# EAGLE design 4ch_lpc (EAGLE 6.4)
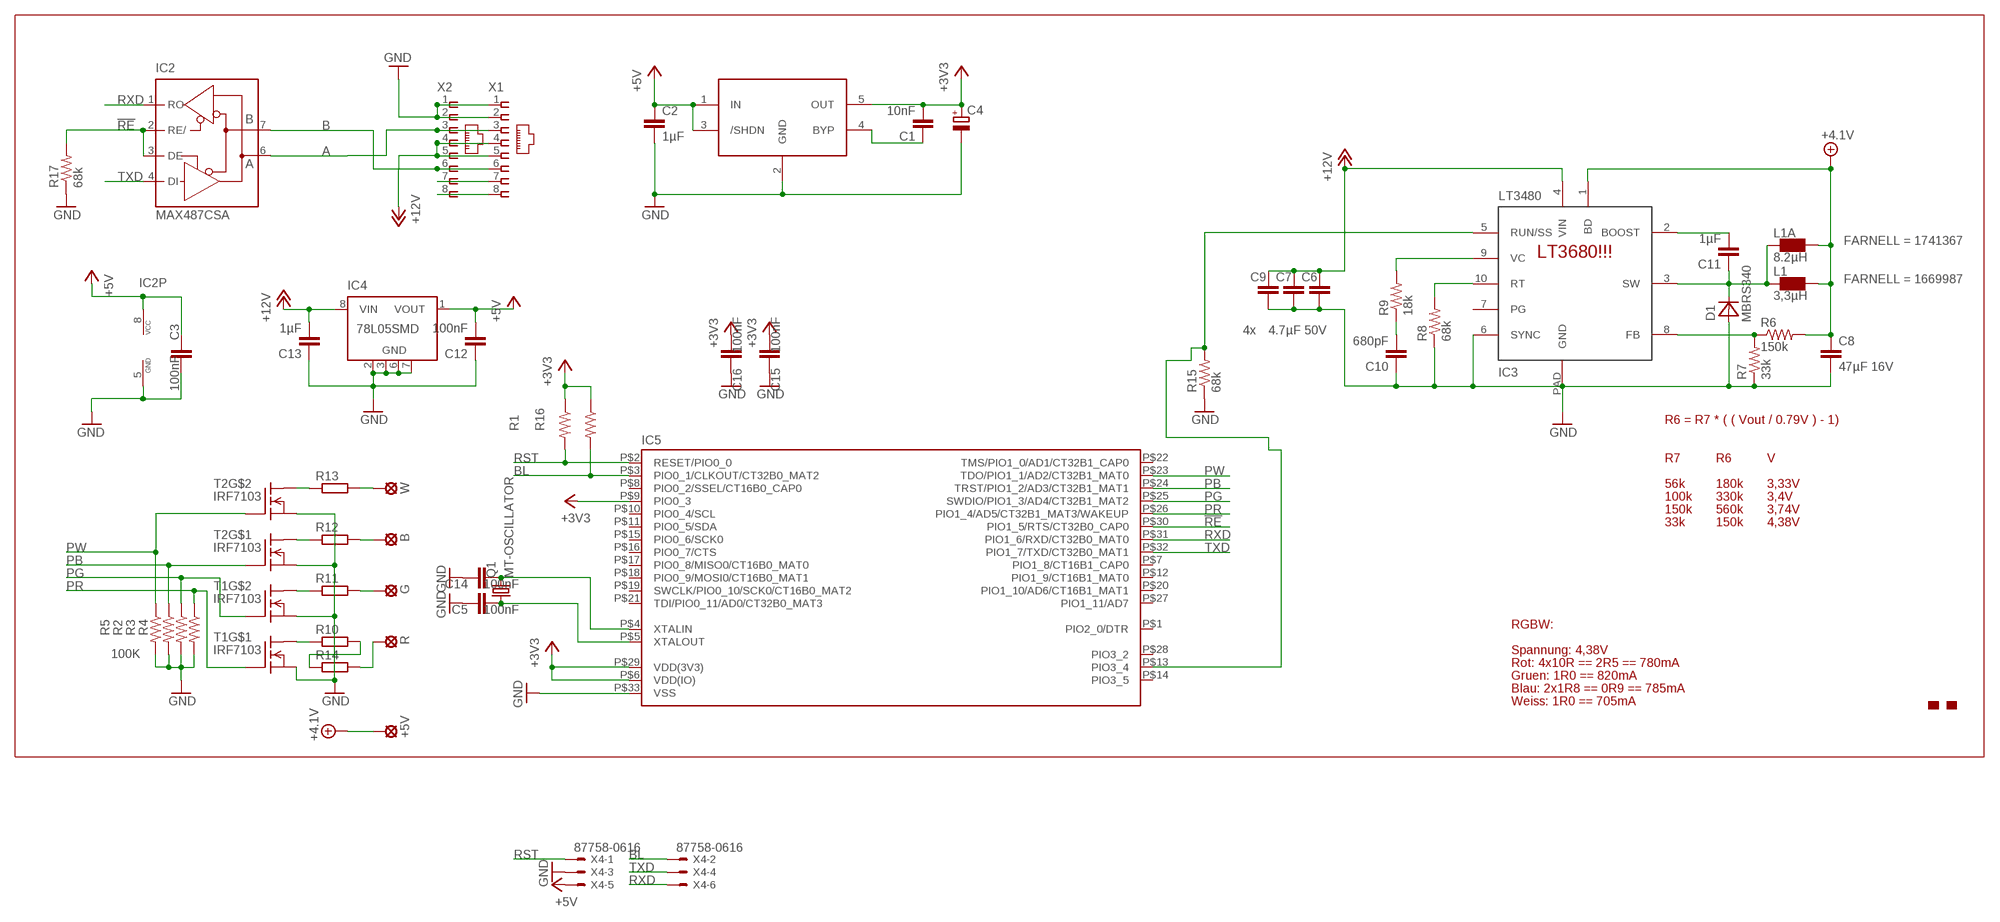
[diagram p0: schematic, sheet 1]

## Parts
+5V  SE14  [SE14]
B  SE14  [SE14]
C1  10nF  C-EUC0402  [C0402]
C2  1µF  CAP0805  [0805]
C3  100nF  CAP0402-CAP  [0402-CAP]
C4  CPOL-EUSMCA  [SMC_A]
C5  100nF  CAP0402-CAP  [0402-CAP]
C6  4.7µF 50V  CAP1210  [1210]
C7  4.7µF 50V  CAP1210  [1210]
C8  47µF 16V  CAP1210  [1210]
C9  4.7µF 50V  CAP1210  [1210]
C10  680pF  CAP0805  [0805]
C11  1µF  CAP0805  [0805]
C12  100nF  CAP0402-CAP  [0402-CAP]
C13  1µF  CAP0805  [0805]
C14  100nF  CAP0402-CAP  [0402-CAP]
C15  100nF  CAP0402-CAP  [0402-CAP]
C16  100nF  CAP0402-CAP  [0402-CAP]
D1  MBRS340  [DO214AB]
G  SE14  [SE14]
IC1  LT1761  [SOT23-5L]
IC2  MAX487CSA  MAX481CSA  [SO08]
IC3  LT3972  LT3480  [MSOP10-PAD]
IC4  78L05SMD  [SO08]
IC5  LPC1113/4_QFN  [HVQFN33-7X7]
L1  3,3µH  TDK_RLF7030  [RLF7030]
L1A  8.2µH  IHLP-2525CZ  [IHLP-2525CZ]
Q1  MT-OSCILLATOR  [MT]
R  SE14  [SE14]
R1  100K  RESISTOR0402-RES  [0402-RES]
R2  100K  RESISTOR0402-RES  [0402-RES]
R3  100K  RESISTOR0402-RES  [0402-RES]
R4  100K  RESISTOR0402-RES  [0402-RES]
R5  100K  RESISTOR0402-RES  [0402-RES]
R6  150k  RESISTOR0805-RES  [0805]
R7  33k  RESISTOR0805-RES  [0805]
R8  68k  RESISTOR0805-RES  [0805]
R9  18k  RESISTOR0805-RES  [0805]
R10  R-EU_MELF0207R  [MINI_MELF-0207R]
R11  R-EU_MELF0207R  [MINI_MELF-0207R]
R12  R-EU_MELF0207R  [MINI_MELF-0207R]
R13  R-EU_MELF0207R  [MINI_MELF-0207R]
R14  R-EU_MELF0207R  [MINI_MELF-0207R]
R15  68k  RESISTOR0402-RES  [0402-RES]
R16  100K  RESISTOR0402-RES  [0402-RES]
R17  68k  RESISTOR0402-RES  [0402-RES]
T1  IRF7103  [SO-8]
T2  IRF7103  [SO-8]
U$1  MAKE-DD_LOGO'PROMPT'  [MAKE-DD_LOGO_PROMPT]
W  SE14  [SE14]
X1  RJ45-8L-B  [RJ45-NO-SHIELD]
X2  RJ45-8L-B  [RJ45-NO-SHIELD]
X4  87758-0616  [87758-0616]

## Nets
!RE: IC2.2(RE/) IC2.3(DE) IC5.P$30(PIO1_5/RTS/CT32B0_CAP0) R17.2
+3V3: C1.2 C4.+ C15.2 C16.2 IC1.5(OUT) IC5.P$6(VDD(IO)) IC5.P$9(PIO0_3) IC5.P$29(VDD(3V3)) R1.1 R16.1
+4.1V: +5V.MP C8.1 IC3.1(BD) L1.P$1 L1A.P$1 R6.2
+5V: C2.1 C3.1 C12.2 IC1.1(IN) IC1.3(/SHDN) IC2.8(VCC) IC4.1(VOUT) X4.5
+12V: C6.1 C7.1 C9.1 C13.2 IC3.4(VIN) IC4.8(VIN) X1.4 X1.5 X2.4 X2.5
A: IC2.6(A) X1.3 X2.3
B: IC2.7(B) X1.6 X2.6
BL: IC5.P$3(PIO0_1/CLKOUT/CT32B0_MAT2) R16.2 X4.2
GND: C2.2 C3.2 C4.- C5.1 C6.2 C7.2 C8.2 C9.2 C10.1 C12.1 C13.1 C14.1 C15.1 C16.1 D1.A IC1.2(GND) IC2.5(GND) IC3.6(SYNC) IC3.PAD(GND) IC4.2(GND) IC4.3(GND) IC4.6(GND) IC4.7(GND) IC5.P$33(VSS) R2.2 R3.2 R4.2 R5.2 R7.1 R8.1 R15.1 R17.1 T1.1(S) T1.3(S) T2.1(S) T2.3(S) X1.1 X1.2 X2.1 X2.2 X4.3
N$1: R10.1 T1.8(D1)
N$2: R13.2 W.MP
N$3: R13.1 T2.5(D1)
N$4: R11.1 T1.5(D1)
N$5: R12.1 T2.8(D1)
N$6: IC3.10(RT) R8.2
N$7: C1.1 IC1.4(BYP)
N$8: G.MP R11.2
N$9: B.MP R12.2
N$10: C10.2 R9.1
N$11: R10.2 R14.1
N$12: IC3.5(RUN/SS) IC5.P$13(PIO3_4) R15.2
N$13: R14.2 R.MP
N$14: IC3.9(VC) R9.2
N$15: C11.1 D1.K(C) IC3.3(SW) L1.P$2 L1A.P$2
N$16: IC3.8(FB) R6.1 R7.2
N$17: C11.2 IC3.2(BOOST)
N$18: X1.7 X2.7
N$19: X1.8 X2.8
N$20: C5.2 IC5.P$5(XTALOUT) Q1.1
N$21: C14.2 IC5.P$4(XTALIN) Q1.3
PB: IC5.P$24(TRST/PIO1_2/AD3/CT32B1_MAT1) R2.1 T2.2(G)
PG: IC5.P$25(SWDIO/PIO1_3/AD4/CT32B1_MAT2) R3.1 T1.4(G)
PR: IC5.P$26(PIO1_4/AD5/CT32B1_MAT3/WAKEUP) R4.1 T1.2(G)
PW: IC5.P$23(TDO/PIO1_1/AD2/CT32B1_MAT0) R5.1 T2.4(G)
RST: IC5.P$2(RESET/PIO0_0) R1.2 X4.1
RXD: IC2.1(RO) IC5.P$31(PIO1_6/RXD/CT32B0_MAT0) X4.6
TXD: IC2.4(DI) IC5.P$32(PIO1_7/TXD/CT32B0_MAT1) X4.4
Unconnected: IC3.7(PG) IC4.4(NC) IC4.5(NC) IC5.P$1(PIO2_0/DTR) IC5.P$7(PIO1_8/CT16B1_CAP0) IC5.P$8(PIO0_2/SSEL/CT16B0_CAP0) IC5.P$10(PIO0_4/SCL) IC5.P$11(PIO0_5/SDA) IC5.P$12(PIO1_9/CT16B1_MAT0) IC5.P$14(PIO3_5) IC5.P$15(PIO0_6/SCK0) IC5.P$16(PIO0_7/CTS) IC5.P$17(PIO0_8/MISO0/CT16B0_MAT0) IC5.P$18(PIO0_9/MOSI0/CT16B0_MAT1) IC5.P$19(SWCLK/PIO0_10/SCK0/CT16B0_MAT2) IC5.P$20(PIO1_10/AD6/CT16B1_MAT1) IC5.P$21(TDI/PIO0_11/AD0/CT32B0_MAT3) IC5.P$22(TMS/PIO1_0/AD1/CT32B1_CAP0) IC5.P$27(PIO1_11/AD7) IC5.P$28(PIO3_2) T1.6(D) T1.7(D) T2.6(D) T2.7(D)

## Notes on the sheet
- LT3680!!!
- 4x
- R6 = R7 * ( ( Vout / 0.79V ) - 1)
- R7 | R6 | V
- 56k | 180k | 3,33V
- 100k | 330k | 3,4V
- 150k | 560k | 3,74V
- 33k | 150k | 4,38V
- RGBW:
- Spannung: 4,38V
- Rot: 4x10R == 2R5 == 780mA
- Gruen: 1R0 == 820mA
- Blau: 2x1R8 == 0R9 == 785mA
- Weiss: 1R0 == 705mA

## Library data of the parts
+5V B G R W = solpad:SE14: SOLDER PAD
C1 = rcl:C-EU: CAPACITOR, European symbol
C2 = SparkFun-Capacitors:CAP: Capacitor
C3 C5-C16 = SparkFun:CAP: Capacitor
C4 = rcl:CPOL-EU: POLARIZED CAPACITOR, European symbol
D1 = seb:MBRS340
IC1 = seb:LT1761
IC2 = maxim:MAX481CSA: RS485 TRANSEIVER; MF: MAXIM; MPN: MAX481CSA; OC_FARNELL: unknown; OC_NEWARK: 90C3817
IC3 = seb:LT3480
IC4 = linear:78L*SMD: Positive VOLTAGE REGULATOR
IC5 = microbuilder:LPC1113/4_QFN: LPC1113/4 ARM Cortex-M0 processor, running at frequencies of up to 50 MHz. QFN 33 Pin Package; DIGIKEY#: 568-4948-ND; MANF: NXP; MANF#: LPC1114FHN33/301,5
L1 = seb:TDK_RLF7030; FARNELL: 1669987
L1A = seb:IHLP-2525CZ; FARNELL: 1741367
Q1 = seb:MT-OSCILLATOR
R1-R9 R15-R17 = SparkFun:RESISTOR: Resistor
R10-R14 = rcl:R-EU_: RESISTOR, European symbol
T1 T2 = transistor-fet+irf7201:IRF7103
U$1 = seb:MAKE-DD_LOGO
X1 X2 = con-tycoelectronics:RJ45: CORCOM Modular RJ Jacks No Shield Source: www.tycoelectronics.com .. ENG_DS_1654001_1099_RJ_L_0507.pdf; MF: TYCO ELECTRONICS; MPN: RJ45-8L-B; OC_FARNELL: 1279843; OC_NEWARK: 52K4445
X4 = con-molex:87758-0616: 6 Pin - 2mm Dual Row Single Wafer, Vertical T/H HDR Source: http://www.molex.com/pdm_docs/sd/877580616_sd.pdf; MPN: 87758-0616; OC_FARNELL: 7472323; OC_NEWARK: 25M5667

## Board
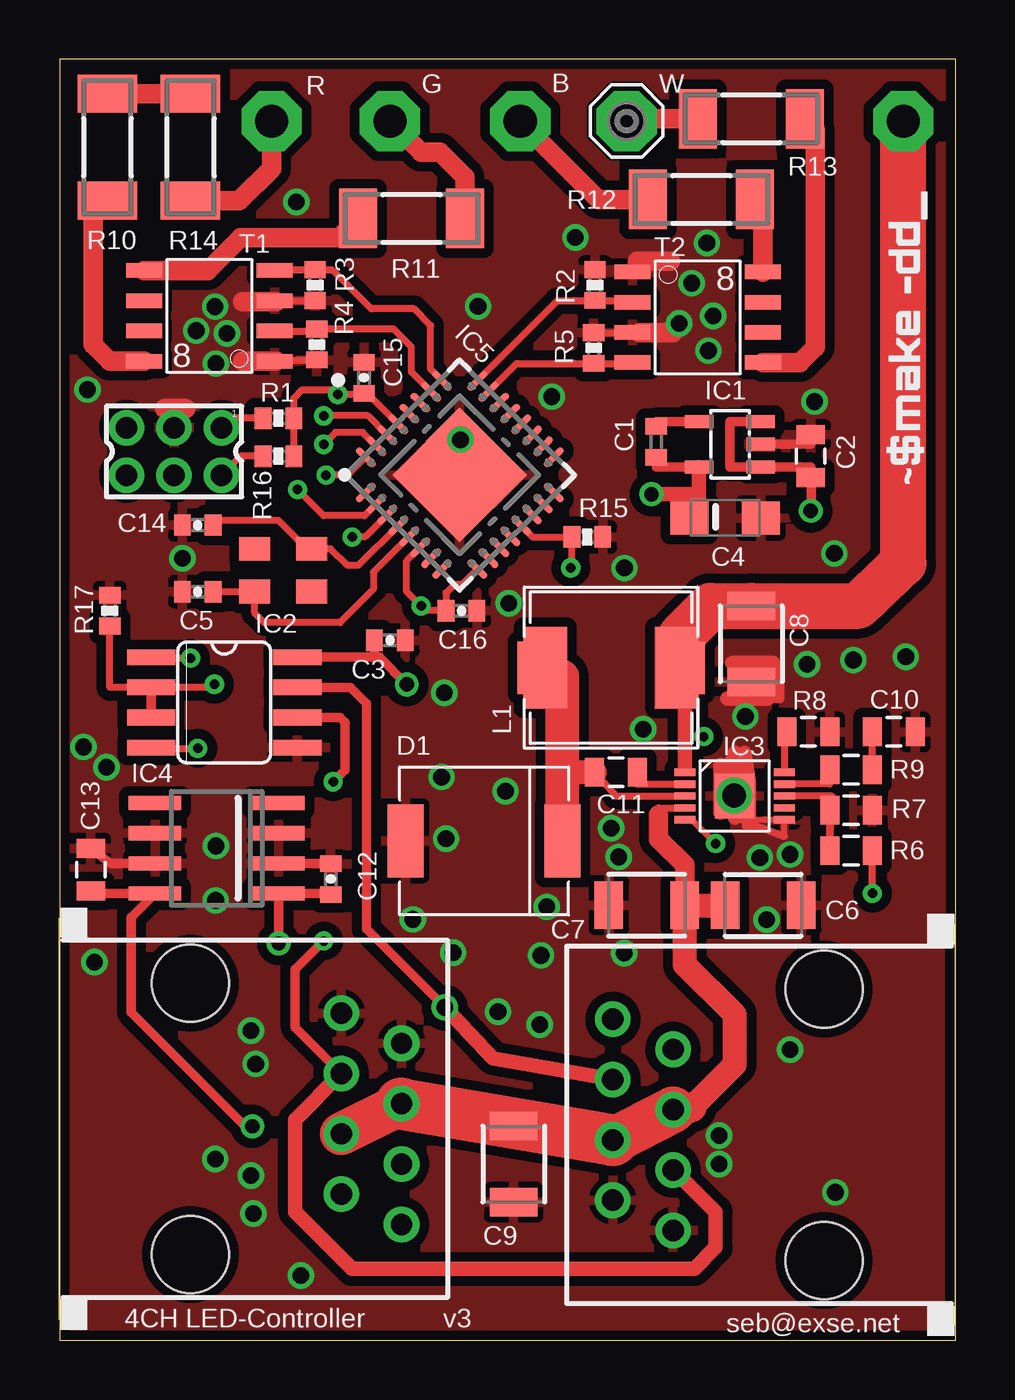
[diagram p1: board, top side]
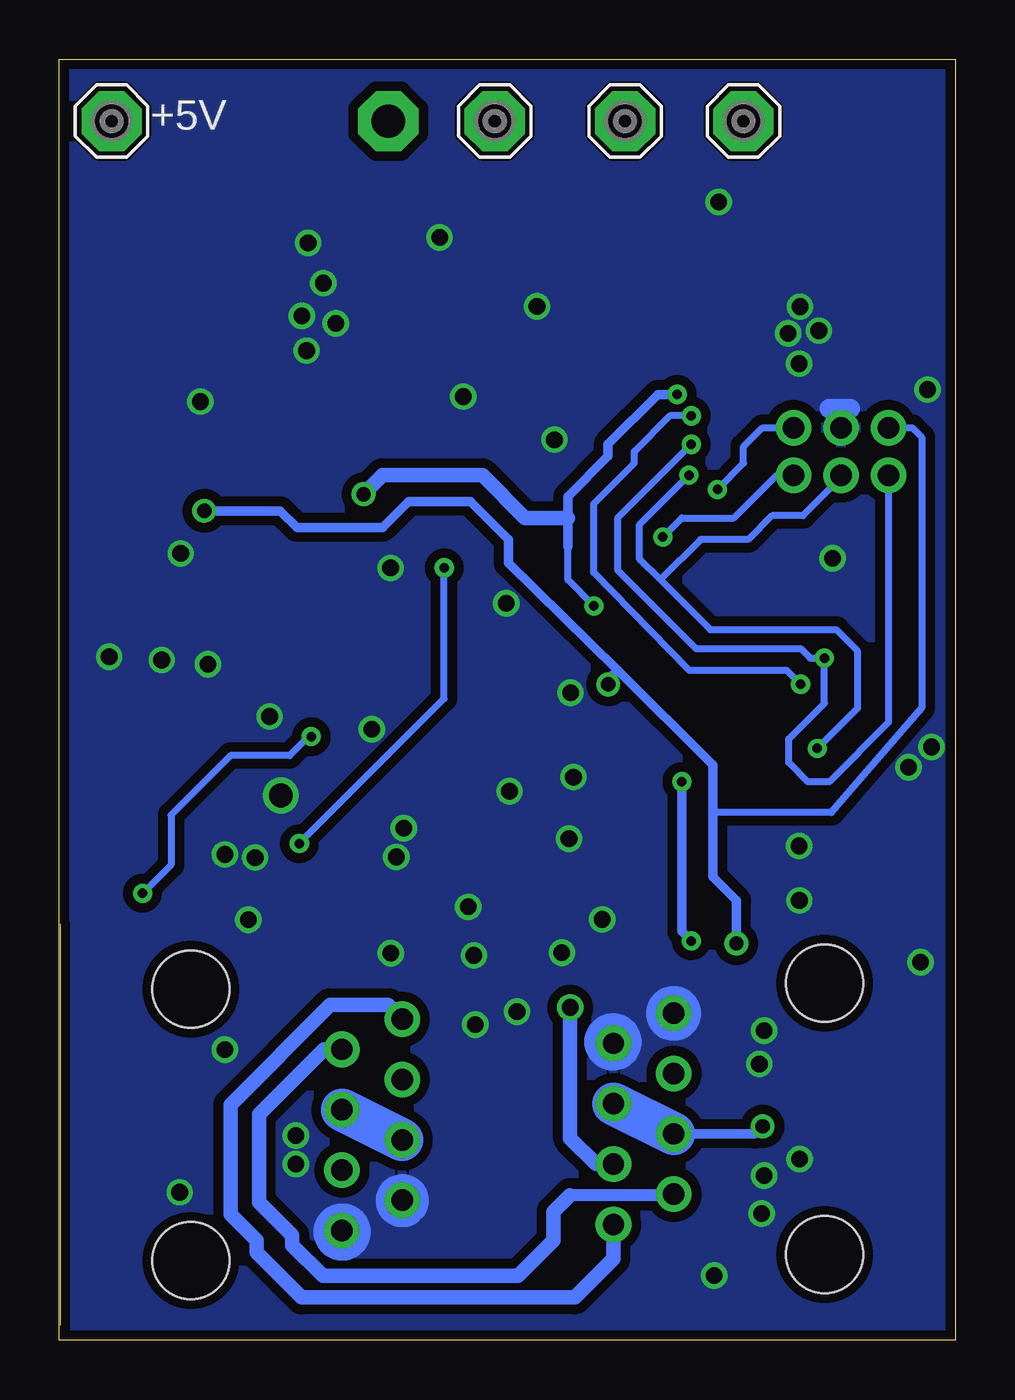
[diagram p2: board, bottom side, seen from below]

Size 37.72 x 53.9 mm. Coordinates in mm from the lower left corner, seen from the top.
Outline: 0.02,0 37.72,0 37.72,53.9 0.02,53.9 0.02,0
Copper layers (1*16): Top 0.035mm / dielectric 1.5mm / Bottom 0.035mm
Design rules "default *": minimum track width 0.2mm, minimum drill 0.4mm, track to track 0.2mm, track to pad 0.2mm, pad to pad 0.2mm, via to via 0.2mm, smd to smd 0mil, copper to edge 0.4mm, drill to drill 8mil, minimum pad ring 0.3mm, minimum via ring 8mil, stop-mask expansion 4mil, vias tented up to drill 40mil, thermal gap 10mil

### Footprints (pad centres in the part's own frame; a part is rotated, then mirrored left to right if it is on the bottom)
SE14 = drill 1.397 pad 2.54 octagon: MP 0,0
C0402 = smd 0.7 x 0.9: 1 -0.65,0; 2 0.65,0
0805 = smd 0.8 x 1.2: 1 -0.9,0; 2 0.9,0
0402-CAP = smd 0.7 x 0.9: 1 -0.65,0; 2 0.65,0
SMC_A = smd 1.6 x 1.4: + -1.5,0; - 1.5,0
1210 = smd 1.2 x 2: 1 -1.6,0; 2 1.6,0
DO214AB = smd 1.52 x 3.07: A 3.305,0; K -3.305,0
SOT23-5L = smd 0.55 x 1.2: 1 -0.95,-1.3; 2 0,-1.3; 3 0.95,-1.3; 4 0.95,1.3; 5 -0.95,1.3
SO08 = smd 0.66 x 2.032: 1 -1.905,-3.073; 2 -0.635,-3.073; 3 0.635,-3.073; 4 1.905,-3.073; 5 1.905,3.073; 6 0.635,3.073; 7 -0.635,3.073; 8 -1.905,3.073
MSOP10-PAD = smd 0.305 x 0.889: 1 -1,-2.095; 2 -0.5,-2.095; 3 0,-2.095; 4 0.5,-2.095; 5 1,-2.095; 6 1,2.095; 7 0.5,2.095; 8 0,2.095; 9 -0.5,2.095; 10 -1,2.095 | smd 1.88 x 1.68: PAD 0,0
SO08' = smd 0.6 x 2.2: 1 -1.905,-2.6; 2 -0.635,-2.6; 3 0.635,-2.6; 4 1.905,-2.6; 5 1.905,2.6; 6 0.635,2.6; 7 -0.635,2.6; 8 -1.905,2.6
HVQFN33-7X7 = smd 1.067 x 0.3: P$1 -3.327,2.275; P$2 -3.327,1.625; P$3 -3.327,0.975; P$4 -3.327,0.325; P$5 -3.327,-0.325; P$6 -3.327,-0.975; P$7 -3.327,-1.625; P$8 -3.327,-2.275; P$17 3.327,-2.275; P$18 3.327,-1.625; P$19 3.327,-0.975; P$20 3.327,-0.325; P$21 3.327,0.325; P$22 3.327,0.975; P$23 3.327,1.625; P$24 3.327,2.275 | smd 0.3 x 1.067: P$9 -2.275,-3.327; P$10 -1.625,-3.327; P$11 -0.975,-3.327; P$12 -0.325,-3.327; P$13 0.325,-3.327; P$14 0.975,-3.327; P$15 1.625,-3.327; P$16 2.275,-3.327; P$25 2.275,3.327; P$26 1.625,3.327; P$27 0.975,3.327; P$28 0.325,3.327; P$29 -0.325,3.327; P$30 -0.975,3.327; P$31 -1.625,3.327; P$32 -2.275,3.327 | smd 4 x 4: P$33 0,0
RLF7030 = smd 2 x 2.2: P$1 -2.95,0; P$2 2.95,0
IHLP-2525CZ = smd 1.83 x 3.43: P$1 -2.77,0; P$2 2.77,0
MT = smd 1.3 x 1: 1 1.2,0.9; 2 -1.2,0.9; 3 -1.2,-0.9; 4 1.2,-0.9
0402-RES = smd 0.7 x 0.9: 1 -0.65,0; 2 0.65,0
MINI_MELF-0207R = smd 1.6 x 2.5: 1 -2.25,0; 2 2.25,0
SO-8 = smd 1.524 x 0.61: 1 -2.743,1.27; 2 -2.743,0; 3 -2.743,-1.27; 4 -2.743,-2.54; 5 2.743,-2.54; 6 2.743,-1.27; 7 2.743,0; 8 2.743,1.27
RJ45-NO-SHIELD = drill 0.9 pad 1.4: 1 -4.445,6.35; 2 -3.175,8.89; 3 -1.905,6.35; 4 -0.635,8.89; 5 0.635,6.35; 6 1.905,8.89; 7 3.175,6.35; 8 4.445,8.89 | hole 3.251: -5.715,0; 5.715,0
87758-0616 = drill 0.9 pad 1.27: 1 -2,-1; 2 -2,1; 3 0,-1; 4 0,1; 5 2,-1; 6 2,1

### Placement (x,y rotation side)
+5V  35.52,51.3 0 bottom
B  19.39,51.3 0 bottom
C1  25.12,37.8 270 top
C2  31.62,37.2 90 top
C3  13.91,29.45 0 top
C4  28.02,34.6 0 top
C5  5.82,31.5 0 top
C6  29.62,18.3 0 top
C7  24.72,18.3 180 top
C8  29.12,29.3 270 top
C9  19.12,7.4 270 top
C10  35.12,25.6 180 top
C11  23.42,23.9 0 top
C12  11.42,19.4 270 top
C13  1.32,19.8 270 top
C14  5.82,34.3 0 top
C15  12.82,40.5 270 top
C16  16.92,30.7 180 top
D1  17.87,21.01 180 top
G  13.91,51.3 0 bottom
IC1  28.22,37.7 90 top
IC2  6.94,26.84 270 top
IC3  28.42,22.9 270 top
IC4  78L05SMD  [SO08']  6.62,20.7 90 top
IC5  16.85,36.41 45 top
L1  23.22,28.3 180 top
L1A  23.22,28.3 180 top
Q1  9.42,32.4 180 top
R  8.93,51.3 0 bottom
R1  9.22,38.8 180 top
R2  22.54,44.4 90 top
R3  10.76,44.4 270 top
R4  10.84,41.9 270 top
R5  22.49,41.75 90 top
R6  33.32,20.6 0 top
R7  33.32,22.3 180 top
R8  31.52,25.6 180 top
R9  33.32,24 180 top
R10  2.02,50.2 90 top
R11  14.82,47.2 0 top
R12  27.02,48 180 top
R13  29.12,51.4 180 top
R14  5.52,50.2 270 top
R15  22.22,33.8 180 top
R16  9.22,37.2 180 top
R17  2.12,30.7 270 top
T1  6.31,42.47 180 top
T2  26.87,43.68 0 top
U$1  36.22,36.2 90 top
W  23.88,51.3 0 top
X1  32.18,9.06 90 top
X2  5.51,9.31 270 top
X4  4.82,37.4 180 top

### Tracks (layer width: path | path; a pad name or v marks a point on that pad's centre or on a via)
!RE  (via drill 0.4)
  Top 0.3: IC5.P$30 12.99,38.9 v11.12,38.9
  Top 0.305: v6.52,27.6 6.39,27.47 IC2.2 2.12,27.47 R17.2
  Top 0.406: IC2.3 IC2.2
  Bottom 0.305: v11.12,38.9 12.02,38.9 13.52,37.4 13.52,36.9 15.22,35.2 15.22,32.3 11.22,28.2 7.12,28.2 v6.52,27.6
+3V3  (via drill 0.4, 0.6)
  Top 0.3: IC5.P$6 14.62,32.8 | IC5.P$29 12.95,39.85 C15.2 12.77,39.8 v11.72,39.8 | R16.1 R1.1
  Top 0.305: 14.62,32.8 14.62,31.5 v15.22,30.9 15.42,30.7 C16.2 16.27,31.45 16.62,31.8 16.94,31.8 IC5.P$9 | R1.1 9.87,39.65 10.22,40 11.52,40 v11.72,39.8
  Top 0.406: C1.2 25.12,36.75 IC1.5
  Top 0.61: IC1.5 26.92,35.5 | 26.92,35.5 26.92,34.4 C4.+ | v24.92,35.6 26.82,35.6 26.92,35.5
  Bottom 0.305: v15.22,30.9 16.32,32 16.32,33.4
  Bottom 0.406: v11.72,39.8 12.52,39.8 14.62,37.7 14.62,37.2 16.32,35.5 16.32,34.6 16.32,33.4
  Bottom 0.61: v24.92,35.6 24.12,36.4 19.92,36.4 18.12,34.6 16.32,34.6
+4.1V  (via drill 0.4)
  Top 0.254: L1.P$1 L1A.P$1
  Top 0.305: IC3.1 26.32,24.8 | v34.22,18.8 R6.2 | 26.32,25.4 v27.12,25.4
  Top 0.61: 26.32,24.1 26.32,24.8 26.32,25.4 26.32,27.9 L1.P$1
  Top 1.93: L1.P$1 26.17,29.65 27.42,30.9 C8.1 33.62,30.9 35.52,32.7 +5V.MP
  Bottom 0.305: v34.22,18.8 33.02,20 33.02,22.1 30.52,24.6 28.02,24.6 27.22,25.4 v27.12,25.4
+5V  (via drill 0.6)
  Top 0.406: C12.2 11.32,18.8 IC4.1 v9.22,16.7 | 13.22,28.74 13.48,28.74 v14.62,27.6 | 13.22,28.74 IC2.8 | v31.62,34.9 31.67,36.25 31.62,36.75 | 31.62,36.75 IC1.1 28.22,36.75 28.22,38.65 IC1.3 | C2.1 31.62,36.75 | C3.1 13.26,28.78 13.22,28.74
  Bottom 0.305: X4.5 1.82,38.4 1.42,38 1.42,26.6 5.22,22.2 10.22,22.2
  Bottom 0.406: v9.22,16.7 9.22,18.5 10.22,19.5 10.22,22.2 10.22,24.2 14.22,28.2 | 14.22,28.2 18.82,32.7 18.82,33.7 20.42,35.3 23.02,35.3 24.12,34.2 27.72,34.2 28.42,34.9 v31.62,34.9 | v14.62,27.6 14.62,27.8 14.22,28.2
+12V  (via drill 0.6)
  Top 0.3: IC3.4 25.22,22.4 25.22,22.1
  Top 0.406: v8.12,9 7.82,9 3.02,13.8 3.02,17.8 IC4.8 1.63,18.8 C13.2
  Top 0.813: 25.22,22.1 25.22,21.1 26.32,20 C7.1
  Top 1.016: 26.52,9.7 26.62,9.8 28.42,11.6 28.42,13.7 26.32,15.8 C7.1 C6.1 | C9.1 20.4,8.43 X1.4
  Top 1.27: X1.5 26.62,9.8
  Top 1.778: X2.5 X2.4
  Top 1.93: X1.5 23.32,8.4 X1.5
  Top 2.184: X2.4 X1.4
  Bottom 0.406: v8.12,9 8.44,8.68 X2.5
  Bottom 1.778: X1.4 X1.5 | X2.5 X2.4
A  (via drill 0.4)
  Top 0.406: IC2.6 11.82,26.2 12.02,26 12.02,24 v11.52,23.5 | X2.3 9.92,13.16 9.92,15.6 v11.12,16.8
  Top 0.61: X1.3 25.87,7.16 27.62,5.4 27.62,3.9 26.72,3 12.32,3 9.92,5.4 9.92,9.28 X2.3
  Bottom 0.406: v11.52,23.5 11.52,17.2 v11.12,16.8
B  (via drill 0.7)
  Top 0.406: IC2.7 12.25,27.47 12.92,26.8 12.92,17.3 v16.22,14
  Top 0.61: X1.6 18.26,11.87 v16.22,14
  Bottom 0.61: v16.22,14 16.22,8.5 15.13,7.41 X2.6
BL  (via drill 0.4)
  Top 0.3: IC5.P$3 12.86,33.8 v12.32,33.8
  Top 0.305: R16.2 7.62,37.2 X4.2
  Bottom 0.305: v12.32,33.8 11.52,34.6 9.32,34.6 7.52,36.4 X4.2
GND  (via drill 0.7, 1)
  Top 0.254: 29.23,21.9 IC3.6 30.52,21.2
  Top 0.3: 9.21,41.25 9.16,41.2 T1.1
  Top 0.305: R5.2 T2.3 | T1.3 9.07,43.75 R3.2 | 9.21,41.25 R4.2 | 28.42,22 30.52,21.2 | 5.32,39.2 5.32,39.3 X4.3
  Top 0.406: C13.1 2.16,20.07 IC4.7 | IC4.2 11.49,20.07 C12.1 | 27.82,24.2 28.02,24.2 28.42,24.6 | 30.02,28.5 30.32,28.2 30.32,27 29.82,27 C8.2 | 9.02,41.2 T1.1 | IC1.2 31.62,37.7 C2.2
  Top 0.61: 28.82,24.7 29.02,23.5 29.02,21.7 | 28.42,22 IC3.PAD 28.42,24.6 28.42,24.7 | 27.82,24.2 27.82,22.2 | 29.82,27 28.12,27 | 30.02,28.5 28.32,28.5 | IC5.P$33 16.88,36.44 v16.88,37.9
  Top 0.813: 24.32,45.4 25.72,45.4 | 26.02,42.7 25.82,42.5 25.82,42.4 24.42,42.4 | 7.72,43.7 9.12,43.7 | 7.72,41.2 9.12,41.2 | 5.32,39.2 4.42,39.2
  Bottom 0.305: 5.32,39.2 4.82,39.2 X4.3
  Bottom 0.61: 11.02,13.7 arc353 11.02,13.8 11.82,13.8 X2.1 | 13.52,12.6 arc-354 13.52,12.5 | 24.92,4.6 arc-354 24.92,4.5 | X1.2 22.91,5.5 22.82,5.2 arc340 22.62,5.4
  Bottom 0.813: 5.32,39.2 4.42,39.2
  other vias: 21.72,46.41 27.26,46.18 27.32,41.64 26.62,44.48 27.52,43.11 26.08,42.8 23.78,32.5 31.47,28.44 31.78,39.5 35.63,28.76 33.42,28.62 5.76,42.48 6.55,43.5 7.04,42.36 6.58,41.1 28.87,26.24 29.77,17.69 29.48,20.31 30.76,20.44 1.18,40 1.01,24.96 28.4,22.92 1.97,24.1 6.58,20.8 18.77,23.1 16.21,27.24 6.57,18.5 23.22,21.54 16.08,23.7 16.27,21.11 23.77,16.29 23.54,20.33 14.87,17.71 20.52,18.23 27.77,8.61 27.77,7.41 20.27,16.19 16.57,16.31 18.46,13.82 20.21,13.28 8.06,6.92 6.56,7.62 8.26,11.62 8.06,13.02 10.16,2.72 8.16,5.32 30.76,12.22 32.66,6.22 17.62,43.51 20.72,39.71 18.92,31.01 32.62,33.11 1.47,15.9 24.57,25.7 9.97,47.9 5.17,32.9
  pour Bottom (isolate 0.406, rank 2): 0.06,53.88 0.02,0 37.71,0 37.7,53.88
  pour Top (isolate 0.406, rank 2): 0.04,53.85 0.02,0 37.74,0 37.7,53.88
N$1
  Top 0.813: T1.8 2.12,41.2 1.42,41.9 1.42,47.35 R10.1
N$2
  Top 0.813: R13.2 23.98,51.4 W.MP
N$3
  Top 0.813: T2.5 31.16,41.14 31.82,41.8 31.82,50.95 R13.1
N$4
  Top 0.813: T1.5 6.23,45.01 7.62,46.4 11.77,46.4 R11.1
N$5
  Top 0.813: T2.8 29.61,47.66 R12.1
N$6
  Top 0.305: IC3.10 30.52,25 R8.2
N$7
  Top 0.406: C1.1 25.12,38.65 IC1.4
N$8
  Top 0.813: R11.2 17.07,48.95 16.02,50 15.21,50 G.MP
N$9
  Top 0.813: R12.2 22.69,48 B.MP
N$10
  Top 0.305: R9.1 C10.2
N$11
  Top 0.813: R10.2 R14.1
N$12  (via drill 0.4)
  Top 0.254: IC3.5 26.63,21.9 v27.62,20.9
  Top 0.305: IC5.P$13 19.92,33.8 R15.2 21.57,32.55 v21.52,32.5
  Bottom 0.305: v27.62,20.9 21.52,27 v21.52,32.5
N$13
  Top 0.813: R14.2 7.57,47.95 8.93,49.31 R.MP
N$14
  Top 0.305: IC3.9 32.42,23.4 R9.2
N$15
  Top 0.254: L1.P$2 L1A.P$2
  Top 0.305: IC3.3 23.42,22.9 C11.1
  Top 0.61: D1.K 21.17,23.9
  Top 1.016: 21.17,23.9 C11.1
  Top 1.422: D1.K 21.17,27.92 L1.P$2
N$16
  Top 0.3: R6.1 R7.2
  Top 0.305: IC3.8 32.52,22.9 R6.1
N$17
  Top 0.305: IC3.2 24.32,23.4 C11.2
N$18
  Bottom 0.5: 11.9,6.1 16.22,6.1
  Bottom 0.61: X1.7 26.59,12.23 29.32,9.5 29.32,5.8 27.92,4.4 27.92,4 26.62,2.7 18.42,2.7 16.92,4.2 16.92,5.4 16.22,6.1 | X2.7 11.9,6.1
N$19
  Bottom 0.61: X1.8 23.89,14.1 26.32,14.1 30.52,9.9 30.52,5.3 29.42,4.2 29.42,3.7 27.52,1.8 16.02,1.8 14.4,3.42 X2.8
N$20
  Top 0.3: IC5.P$5 13.22,32.32 13.22,31.6 11.82,30.2 8.62,30.2 8.22,30.6 Q1.1 C5.2
N$21
  Top 0.3: IC5.P$4 12.58,32.6 12.12,32.6 11.42,33.3 Q1.3 10.42,33.3 9.22,34.5 6.52,34.5 C14.2
PB
  Top 0.3: IC5.P$24 20.97,43.75 R2.1
  Top 0.305: T2.2 24.05,43.75 R2.1 21.67,43.75
PG
  Top 0.3: IC5.P$25 15.62,40.86 15.62,42.7 14.92,43.4 13.12,43.4
  Top 0.305: 13.12,43.4 11.47,45.05 R3.1 9.1,45.05 T1.4
PR
  Top 0.3: IC5.P$26 14.82,40.74 14.82,41.8 14.07,42.55 R4.1
  Top 0.305: 10.98,42.4 R4.1 10.76,42.47 T1.2
PW
  Top 0.3: IC5.P$23 19.24,41.1 R5.1
  Top 0.305: T2.4 24.09,41.1 R5.1 21.72,41.1
RST  (via drill 0.4)
  Top 0.3: IC5.P$2 12.84,34.7 11.12,34.7 v10.02,35.8
  Top 0.305: R1.2 7.22,38.8 X4.1
  Bottom 0.305: v10.02,35.8 8.92,36.9 8.92,37.6 8.12,38.4 X4.1
RXD  (via drill 0.4)
  Top 0.3: IC5.P$31 12.77,38.2 11.62,38.2
  Top 0.305: v5.52,28.7 3.91,28.7 IC2.1 | v11.12,37.7 11.62,38.2
  Bottom 0.305: v11.12,37.7 14.22,34.6 14.22,32.4 10.92,29.1 6.52,29.1 6.12,28.7 v5.52,28.7 5.52,26.8 7.02,25.3 7.02,24.3 6.22,23.5 5.32,23.5 2.82,26 X4.6
TXD  (via drill 0.4)
  Top 0.3: IC5.P$32 12.13,36.4 v11.22,36.4
  Top 0.305: v5.82,24.9 3.9,24.9 IC2.4
  Bottom 0.305: v5.82,24.9 4.12,26.6 4.12,29 5.02,29.9 10.32,29.9 12.42,32 | v11.22,36.4 13.32,34.3 13.32,32.9 12.42,32 | X4.4 4.82,36.3 6.42,34.7 7.72,34.7 8.72,33.7 10.72,33.7 12.42,32

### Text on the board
tPlace: seb@exse.net | 4CH LED-Controller | v3
_tNames: R | G | B | W | R13 | R12 | R10 | R14 | R11 | R2 | T2 | R3 | R4 | R5 | T1 | C2 | C3 | C5 | Q1 | R1 | ISP | C4 | IC1 | C8 | IC2 | C1 | R15 | L1 | C10 | R8 | D1 | IC3 | IC4 | C11 | R9 | R7 | C13 | C12 | R6 | C7 | C6 | C9
_bNames: +5V
_tValues: SE14 | 100K | MEGA48/88/168-AU | 3,3µH | 8.2µH | 47µF 16V | 68k | 68k | 680pF | MBRS340 | 18k | 78L05SMD | 33k | 1µF | 1µF | 100nF | LT3972 | 4.7µF 50V | 150k | 4.7µF 50V | RJ45-8L-B | 4.7µF 50V | RJ45-8L-B

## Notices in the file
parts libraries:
microbuilder: This work is placed in the public domain, and may be freely used for commercial and non-commercial work with the following conditions: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
SparkFun-Capacitors: Licensing: CC v3.0 Share-Alike You are welcome to use this library for commercial purposes.
